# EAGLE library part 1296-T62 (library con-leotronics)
1.27mm SINGLE ROW FEMALE SOCKET Source: http://www.leotronics.co.uk/Conexcon/Data%20Sheets/sec.%20A/1296ing.pdf
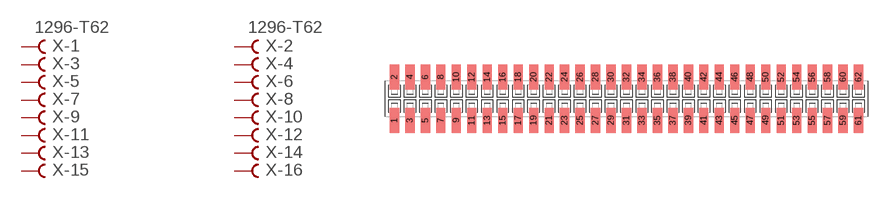
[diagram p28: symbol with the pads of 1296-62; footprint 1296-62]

Designator prefix X; gates -1=FVAL -2=FVAL -3=F -4=F -5=F -6=F -7=F -8=F -9=F -10=F -11=F -12=F -13=F -14=F -15=F -16=F -17=F -18=F -19=F -20=F -21=F -22=F -23=F -24=F -25=F -26=F -27=F -28=F -29=F -30=F -31=F -32=F -33=F -34=F -35=F -36=F -37=F -38=F -39=F -40=F -41=F -42=F -43=F -44=F -45=F -46=F -47=F -48=F -49=F -50=F -51=F -52=F -53=F -54=F -55=F -56=F -57=F -58=F -59=F -60=F -61=F -62=F

## 1296-T62 (OC_FARNELL: unknown; OC_NEWARK: unknown)  [1296-62]
1  -1:B  pas
2  -2:B  pas
3  -3:B  pas
4  -4:B  pas
5  -5:B  pas
6  -6:B  pas
7  -7:B  pas
8  -8:B  pas
9  -9:B  pas
10  -10:B  pas
11  -11:B  pas
12  -12:B  pas
13  -13:B  pas
14  -14:B  pas
15  -15:B  pas
16  -16:B  pas
17  -17:B  pas
18  -18:B  pas
19  -19:B  pas
20  -20:B  pas
21  -21:B  pas
22  -22:B  pas
23  -23:B  pas
24  -24:B  pas
25  -25:B  pas
26  -26:B  pas
27  -27:B  pas
28  -28:B  pas
29  -29:B  pas
30  -30:B  pas
31  -31:B  pas
32  -32:B  pas
33  -33:B  pas
34  -34:B  pas
35  -35:B  pas
36  -36:B  pas
37  -37:B  pas
38  -38:B  pas
39  -39:B  pas
40  -40:B  pas
41  -41:B  pas
42  -42:B  pas
43  -43:B  pas
44  -44:B  pas
45  -45:B  pas
46  -46:B  pas
47  -47:B  pas
48  -48:B  pas
49  -49:B  pas
50  -50:B  pas
51  -51:B  pas
52  -52:B  pas
53  -53:B  pas
54  -54:B  pas
55  -55:B  pas
56  -56:B  pas
57  -57:B  pas
58  -58:B  pas
59  -59:B  pas
60  -60:B  pas
61  -61:B  pas
62  -62:B  pas

## Footprint 1296-62 (pad centres in mm)
1.27mm SINGLE ROW FEMALE SOCKET Source: http://www.leotronics.co.uk/Conexcon/Data%20Sheets/sec.%20A/1296ing.pdf
smd 0.76 x 2.05: 1 -19.05,-1.78; 2 -19.05,1.78; 3 -17.78,-1.78; 4 -17.78,1.78; 5 -16.51,-1.78; 6 -16.51,1.78; 7 -15.24,-1.78; 8 -15.24,1.78; 9 -13.97,-1.78; 10 -13.97,1.78; 11 -12.7,-1.78; 12 -12.7,1.78; 13 -11.43,-1.78; 14 -11.43,1.78; 15 -10.16,-1.78; 16 -10.16,1.78; 17 -8.89,-1.78; 18 -8.89,1.78; 19 -7.62,-1.78; 20 -7.62,1.78; 21 -6.35,-1.78; 22 -6.35,1.78; 23 -5.08,-1.78; 24 -5.08,1.78; 25 -3.81,-1.78; 26 -3.81,1.78; 27 -2.54,-1.78; 28 -2.54,1.78; 29 -1.27,-1.78; 30 -1.27,1.78; 31 0,-1.78; 32 0,1.78; 33 1.27,-1.78; 34 1.27,1.78; 35 2.54,-1.78; 36 2.54,1.78; 37 3.81,-1.78; 38 3.81,1.78; 39 5.08,-1.78; 40 5.08,1.78; 41 6.35,-1.78; 42 6.35,1.78; 43 7.62,-1.78; 44 7.62,1.78; 45 8.89,-1.78; 46 8.89,1.78; 47 10.16,-1.78; 48 10.16,1.78; 49 11.43,-1.78; 50 11.43,1.78; 51 12.7,-1.78; 52 12.7,1.78; 53 13.97,-1.78; 54 13.97,1.78; 55 15.24,-1.78; 56 15.24,1.78; 57 16.51,-1.78; 58 16.51,1.78; 59 17.78,-1.78; 60 17.78,1.78; 61 19.05,-1.78; 62 19.05,1.78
